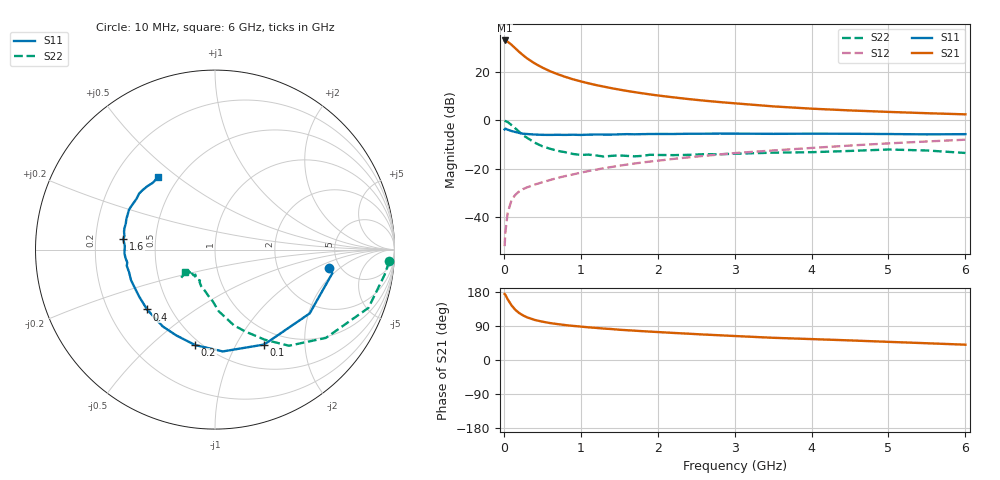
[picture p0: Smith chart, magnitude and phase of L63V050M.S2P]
!  INFINEON TECHNOLOGIES Small Signal Semiconductors
! BFR380L3 , Si-NPN RF-Transistor in TSLP-3-1
!  Vce=3 V,  Ic=50 mA
! Common Emitter S-Parameters:  07. March 2005
#  GHz  S  MA  R  50
! f  S11  S21  S12  S22
! GHz  Mag  Ang  Mag  Ang  Mag  Ang  Mag  Ang
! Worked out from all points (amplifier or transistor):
!   36 points, 10 MHz to 6 GHz, reference 50 ohm
!   highest |S21| = 32.9 dB at 10 MHz (marker M1)
!   |S21| within 3 dB of that: start of sweep to 141.2 MHz
!   unconditionally stable (mu >= 1): 1.562 GHz to 4.828 GHz
!   at 250 MHz: K = 0.49, MSG = 27.6 dB, |S12| = -28.5 dB
!   at 1.4 GHz: K = 0.99, MSG = 16.3 dB, |S12| = -19.4 dB
!   at 6 GHz: K = 0.98, MSG = 5.2 dB, |S12| = -8.1 dB
!   S11 on the Smith chart (normalised r, x): 10 MHz: 4.06, -1.46; 100 MHz: 0.80, -1.31; 200 MHz: 0.47, -0.70; 400 MHz: 0.37, -0.33; 1.6 GHz: 0.32, +0.05; 6 GHz: 0.39, +0.43
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0.01  0.6439 -9.4  44.15 174.1  0.0025 80.4  0.9728 -3.9
0.02  0.6668 -11.4  43.97 172.0  0.0049 81.8  0.9555 -8.4
0.05  0.6361 -34.0  41.58 160.2  0.0122 77.2  0.9145 -20.8
0.1  0.5957 -62.6  35.95 144.2  0.0224 65.3  0.79 -38.5
0.15  0.569 -85.6  30.34 132.2  0.0288 59.1  0.6759 -52.4
0.2  0.5433 -101.7  25.57 123.8  0.0338 56.7  0.5735 -61.1
0.25  0.5244 -114.5  21.91 117.6  0.0377 54.7  0.4865 -69.7
0.3  0.5177 -124.2  18.94 112.7  0.0408 54.3  0.4347 -76.0
0.4  0.5045 -138.6  14.88 105.8  0.0466 54.4  0.3435 -86.6
0.5  0.4971 -148.1  12.18 101.2  0.0521 56.7  0.2889 -92.4
0.6  0.4954 -155.3  10.24 97.5  0.058 58.2  0.2571 -98.8
0.7  0.4979 -160.1  8.875 94.7  0.0643 59.8  0.2323 -105.0
0.9  0.4998 -169.5  6.958 90.0  0.0757 62.8  0.2002 -115.3
1.1  0.5015 -175.0  5.76 86.2  0.089 64.1  0.1941 -120.9
1.3  0.5031 179.2  4.913 82.9  0.102 65.2  0.1771 -128.2
1.6  0.5142 173.2  4.01 78.6  0.1208 65.9  0.1826 -135.5
2.2  0.5178 163.7  2.959 71.5  0.1582 66.4  0.1894 -137.7
2.8  0.5281 155.2  2.365 65.3  0.1951 66.1  0.1973 -143.5
3.5  0.5208 146.9  1.924 58.6  0.2365 63.9  0.2129 -141.9
4.5  0.5227 140.9  1.587 51.7  0.2987 62.2  0.2312 -140.9
5.5  0.5084 132.8  1.39 44.2  0.3626 58.3  0.2361 -140.3
6  0.5138 127.9  1.317 40.4  0.3948 56.0  0.21 -142.7
